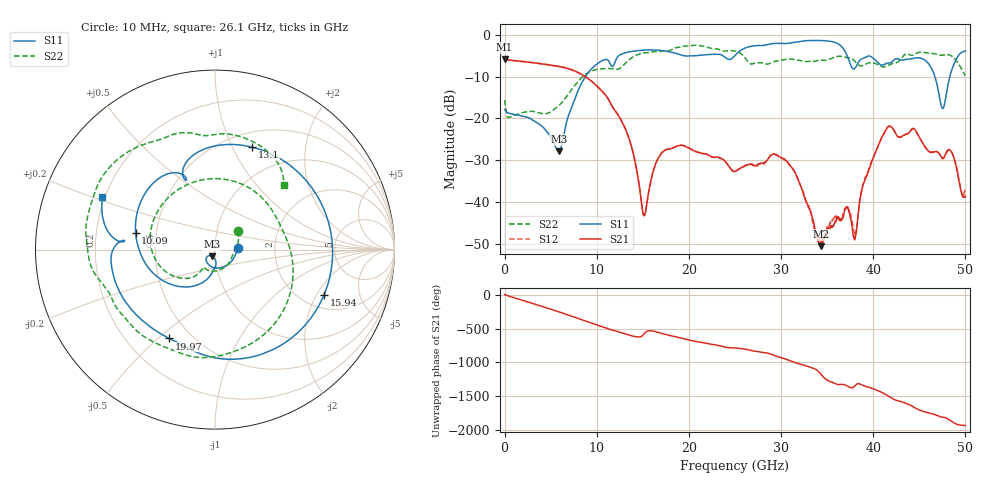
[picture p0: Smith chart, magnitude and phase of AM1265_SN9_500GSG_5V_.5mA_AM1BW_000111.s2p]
!Keysight Technologies,N5245B,MY58422270,A.16.20.02
!Date: Thursday, March 05, 2026 00:30:57
!Correction: S11(C  2-Port  )
!S21(C  2-Port  )
!S12(C  2-Port  )
!S22(C  2-Port  )
!S2P File: Measurements: S11, S21, S12, S22:
# Hz S  dB  R 50
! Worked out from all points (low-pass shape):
!   3201 points, 10 MHz to 50 GHz, reference 50 ohm
!   highest |S21| = -5.84 dB at 10 MHz (marker M1); lowest = -50.5 dB at 34.32 GHz (marker M2)
!   |S21| within 3 dB of the highest: start of sweep to 7.789 GHz
!   lowest |S11| = -27.9 dB at 5.884 GHz (marker M3), VSWR 1.08, Z = 48.1 - j3.52 ohm
!   |S11| at or under -10 dB: start of sweep to 8.786 GHz; 46.69 GHz to 48.31 GHz (1.621 GHz wide, 3.41 % of centre)
!   |S22| runs from -19.8 to -2.5 dB; largest |S21 - S12| = 0.0072
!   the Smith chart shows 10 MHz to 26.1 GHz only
!   S11 on the Smith chart (normalised r, x): 10 MHz: 1.29, +0.02; 10.09 GHz: 0.38, +0.09; 13.1 GHz: 0.66, +1.20; 15.94 GHz: 2.62, -2.32; 19.97 GHz: 0.38, -0.54; 26.1 GHz: 0.19, +0.21
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1e7  -17.87 3.3  -5.84 2.5  -5.85 2.5  -15.58 38.7
2.337659e9  -19.64 -83.6  -6.48 -99.3  -6.48 -99.3  -18.43 -92.5
4.118553e9  -21.94 -127.4  -6.96 -175.0  -6.96 -175.0  -18.84 -121.5
5.883825e9  -27.85 -115.7  -7.57 107.5  -7.57 107.5  -16.97 -123.7
8.352081e9  -11.63 -127.4  -9.47 -7.8  -9.46 -7.7  -10.30 -157.6
1.008611e10  -6.90 168.2  -12.40 -89.2  -12.39 -89.1  -8.26 142.1
1.310113e10  -4.33 70.0  -22.42 141.0  -22.44 140.9  -6.82 -17.5
1.508511e10  -3.69 3.9  -43.13 132.6  -42.88 134.0  -4.31 -102.4
1.594431e10  -3.64 -22.4  -34.15 -174.4  -34.21 -175.0  -4.15 -124.8
1.667854e10  -3.69 -43.7  -29.42 163.0  -29.44 163.2  -4.04 -141.2
1.997476e10  -5.09 -117.2  -27.03 50.5  -26.98 50.8  -2.68 161.4
2.5005e10  -4.97 173.8  -32.65 -66.7  -32.57 -67.2  -3.90 70.8
2.609853e10  -3.19 155.0  -31.26 -84.2  -31.29 -84.5  -5.56 43.4
3.042579e10  -2.11 81.9  -29.91 132.0  -29.75 131.8  -5.92 -47.3
3.334708e10  -1.39 35.6  -43.23 -1.2  -43.72 -3.2  -6.38 -127.7
3.431564e10  -1.39 18.8  -50.48 -93.6  -49.62 -108.5  -6.03 -148.2
3.672141e10  -3.21 -32.1  -43.69 114.2  -42.89 105.1  -5.25 164.6
3.801802e10  -8.03 -26.0  -48.76 94.7  -47.98 94.9  -6.37 139.0
4.167354e10  -6.77 -54.2  -21.83 -59.9  -21.88 -60.0  -7.29 116.1
4.511035e10  -5.58 -102.2  -24.91 91.2  -24.91 91.0  -4.20 75.9
4.770358e10  -16.87 69.8  -29.16 -13.0  -29.35 -12.5  -4.82 40.1
5e10  -3.91 -73.1  -38.53 -131.0  -36.73 -138.6  -9.80 3.1
